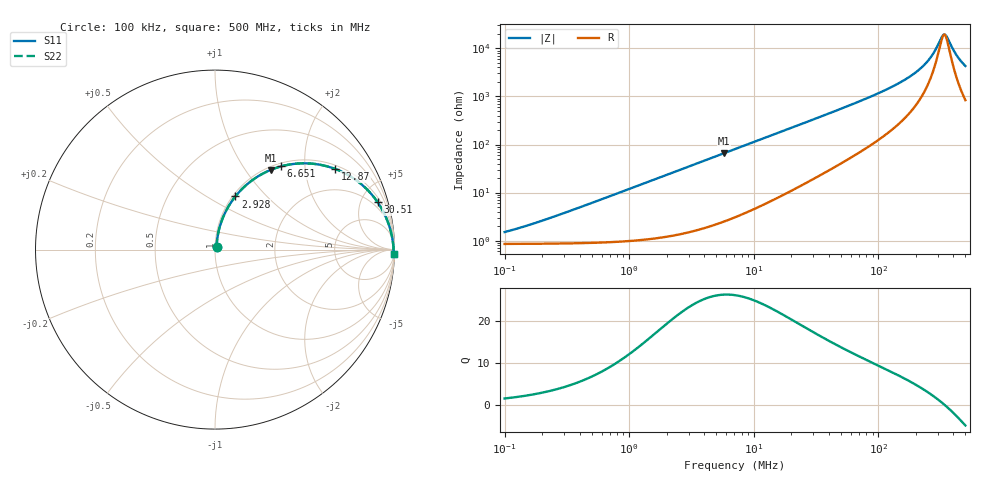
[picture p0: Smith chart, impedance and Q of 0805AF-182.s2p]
# MHz  S  MA  R  50
!Freq  MagS11  AngS11  MagS21  AngS21  MagS12  AngS12  MagS22  AngS22
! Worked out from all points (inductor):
!   801 points, 100 kHz to 500 MHz, reference 50 ohm
!   read as one part in series: L = 1.94 uH near 213.1 kHz
!   highest Q = 26.3 at 5.791 MHz (marker M1), where L = 1.81 uH
!   self-resonance near 335.3 MHz
!   S11 on the Smith chart (normalised r, x): 100 kHz: 1.02, +0.02; 2.928 MHz: 1.03, +0.68; 6.651 MHz: 1.06, +1.51; 12.87 MHz: 1.12, +2.88; 30.51 MHz: 1.39, +6.72; 500 MHz: 18, -84
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0.1  0.01499 54.8  0.9914 -0.7  0.9914 -0.7  0.01499 54.8
0.1758765  0.0231 67.1  0.9912 -1.2  0.9912 -1.2  0.0231 67.1
0.4168304  0.05063 77.1  0.99 -2.9  0.99 -2.9  0.05063 77.1
1.719065  0.1955 75.5  0.9697 -11.3  0.9697 -11.3  0.1955 75.5
2.928332  0.3169 69.1  0.9348 -18.5  0.9348 -18.5  0.3169 69.1
5.790557  0.5414 55.1  0.8205 -32.8  0.8205 -32.8  0.5414 55.1
6.650674  0.592 51.5  0.7837 -36.3  0.7837 -36.3  0.592 51.5
7.089654  0.6153 49.9  0.7652 -37.9  0.7652 -37.9  0.6153 49.9
12.87397  0.8056 34.0  0.5591 -53.6  0.5591 -53.6  0.8056 34.0
19.29843  0.8898 24.5  0.4153 -62.7  0.4153 -62.7  0.8898 24.5
29.55184  0.9411 16.7  0.2886 -70.0  0.2886 -70.0  0.9411 16.7
30.51154  0.9438 16.3  0.2804 -70.4  0.2804 -70.4  0.9438 16.3
58.43654  0.9768 8.6  0.1507 -76.9  0.1507 -76.9  0.9768 8.6
121.8757  0.9896 3.8  0.06697 -79.1  0.06697 -79.1  0.9896 3.8
175.0735  0.9923 2.3  0.03989 -77.8  0.03989 -77.8  0.9923 2.3
226.0778  0.9936 1.3  0.0239 -73.9  0.0239 -73.9  0.9936 1.3
268.0914  0.9943 0.8  0.01429 -66.0  0.01429 -66.0  0.9943 0.8
321.3176  0.9948 0.2  0.00596 -28.5  0.00596 -28.5  0.9948 0.2
335.3055  0.9949 0.0  0.005161 -5.1  0.005161 -5.1  0.9949 0.0
353.6499  0.995 -0.1  0.00564 26.7  0.00564 26.7  0.995 -0.1
423.8626  0.9952 -0.7  0.01372 69.2  0.01372 69.2  0.9952 -0.7
500  0.9952 -1.3  0.02316 77.5  0.02316 77.5  0.9952 -1.3
